FUNCTION_BLOCK "IMAC_TANK_CALL"
TITLE =Function calls for TANK objects
//Parameter Description for Function TANK (FB85):
//-----------------------------------------------
//OBJ:     Ascending Object number for TANK (1...x)
//
//XTsub:    'Substitution Value' for Tank Temperature. The value specified here
//          will be used instaed of the measured value, if the measured value is
//          invalid (Undefined or Out-of-Range or Faded Out or ObjNo invalid).
//          This value is only required, if the density compensation is 'ON' for
//          this tank (see Mode Switch M1_Temperature_Comp).
//          The Unit of XTsub is [°C]
//
//XDensity: 'Density' of the Medium in this tank.
//          This Value can be an input from OS or can be a fixed value.
//          The Unit of XDensity is [kg/dm3] or [tons/m3]
//
//XReftemp: 'Reference Temperature' for given density 'XDensity'.
//          This Value can be an input from OS or can be a fixed value.
//          This value is only required, if the density compensation is 'ON' for
//          this tank (see Mode Switch M1_Temperature_Comp).
//          The Unit of XRefTemp is [°C]
//
//XVEC:     'Volume Expansion Coefficient' - Change of density (staring from
//          XDensity at XReftemp) with every Kelvin of temperature change
//          This Value can be an input from OS or can be a fixed value.
//          This value is only required, if the density compensation is 'ON' for
//          this tank (see Mode Switch M1_Temperature_Comp).
//          The Unit of XVEC is [1/K]
//
//PCONF:    (leave empty, refers to local instance data in Instance DB)
//
//YVolume:  'Computed Volume' of Mediun in the tank
//          The Unit of YVolume is [m3]
//
//YMass:    'Computed Mass' of Mediun in the tank
//          The Unit of YMass is [tons]
//
//YLevel:   'Computed Level' of Mediun in the tank
//          The Unit of YLevel is [m]
//
//OSSTAT:   OS Status Word (not used for TANK)
//
//OSALARM:  OS Alarm Word  (not used for TANK)
//
//
//Units used in FB85 (TANK):
//Pressure MePo        : ................................... [Bar]
//Level MePo           : ................................... [m]
//Volume               : ................................... [m3]
//Temperature MePo     : ................................... [°C]
//Temperature Setpoint : ................................... [°C]
//Density              : ................................... [kg/dm3]
//Mass                 : ................................... [Tons]
//Vol.-Exp.Coefficient : ................................... [1/K]
AUTHOR : Edelmann
FAMILY : IMAC
VERSION : 0.1


VAR
  Tank_No001 : "IMAC_TANK";
  Tank_No002 : "IMAC_TANK";
  Tank_No003 : "IMAC_TANK";
  Tank_No004 : "IMAC_TANK";
  Tank_No005 : "IMAC_TANK";
  Tank_No006 : "IMAC_TANK";
  Tank_No007 : "IMAC_TANK";
  Tank_No008 : "IMAC_TANK";
  Tank_No009 : "IMAC_TANK";
  Tank_No010 : "IMAC_TANK";
END_VAR
BEGIN
NETWORK
TITLE =TANK Number 001

      CALL #Tank_No001 (
           OBJ                      := 1,
           XTsub                    := "IMAC_TANK_I/O".TANK_001_XTsub,// Temperature from OS or fixed value (Substitution Value, if Temp Sensor broken or not available)
           XDensity                 := "IMAC_TANK_I/O".TANK_001_XDensity,// Density from OS or fixed value
           XRefTemp                 := 2.000000e+001,// Reference Temperature for given Density value
           XVEC                     := 0.000000e+000,// Volume Expansion Coefficient from OS or fixed value
           YVolume                  := "IMAC_TANK_I/O".TANK_001_YVolume,// Computed Volume
           YMass                    := "IMAC_TANK_I/O".TANK_001_YMass,// Computed Mass
           YLevel                   := "IMAC_TANK_I/O".TANK_001_YLevel,// Computed Level
           OSSTAT                   := "IMAC_TANK_I/O".TANK_001_OSSTAT,// OS STATUS Word
           OSALARM                  := "IMAC_TANK_I/O".TANK_001_OSALARM);// OS ALARM Word

NETWORK
TITLE =TANK Number 002

//*********** END of function Processing ! *******************************************************************
      BEA   ; // Move this Instruction down to the next Network to add one object !
//************************************************************************************************************

      CALL #Tank_No002 (
           OBJ                      := 2,
           XTsub                    := "IMAC_TANK_I/O".TANK_002_XTsub,// Temperature from OS or fixed value (Substitution Value, if Temp Sensor broken or not available)
           XDensity                 := "IMAC_TANK_I/O".TANK_002_XDensity,// Density from OS or fixed value
           XRefTemp                 := 2.000000e+001,// Reference Temperature for given Density value
           XVEC                     := 0.000000e+000,// Volume Expansion Coefficient from OS or fixed value
           YVolume                  := "IMAC_TANK_I/O".TANK_002_YVolume,// Computed Volume
           YMass                    := "IMAC_TANK_I/O".TANK_002_YMass,// Computed Mass
           YLevel                   := "IMAC_TANK_I/O".TANK_002_YLevel,// Computed Level
           OSSTAT                   := "IMAC_TANK_I/O".TANK_002_OSSTAT,// OS STATUS Word
           OSALARM                  := "IMAC_TANK_I/O".TANK_002_OSALARM);// OS ALARM Word

NETWORK
TITLE =TANK Number 003

      CALL #Tank_No003 (
           OBJ                      := 3,
           XTsub                    := "IMAC_TANK_I/O".TANK_003_XTsub,// Temperature from OS or fixed value (Substitution Value, if Temp Sensor broken or not available)
           XDensity                 := "IMAC_TANK_I/O".TANK_003_XDensity,// Density from OS or fixed value
           XRefTemp                 := 2.000000e+001,// Reference Temperature for given Density value
           XVEC                     := 0.000000e+000,// Volume Expansion Coefficient from OS or fixed value
           YVolume                  := "IMAC_TANK_I/O".TANK_003_YVolume,// Computed Volume
           YMass                    := "IMAC_TANK_I/O".TANK_003_YMass,// Computed Mass
           YLevel                   := "IMAC_TANK_I/O".TANK_003_YLevel,// Computed Level
           OSSTAT                   := "IMAC_TANK_I/O".TANK_003_OSSTAT,// OS STATUS Word
           OSALARM                  := "IMAC_TANK_I/O".TANK_003_OSALARM);// OS ALARM Word

NETWORK
TITLE =TANK Number 004

      CALL #Tank_No004 (
           OBJ                      := 4,
           XTsub                    := "IMAC_TANK_I/O".TANK_004_XTsub,// Temperature from OS or fixed value (Substitution Value, if Temp Sensor broken or not available)
           XDensity                 := "IMAC_TANK_I/O".TANK_004_XDensity,// Density from OS or fixed value
           XRefTemp                 := 2.000000e+001,// Reference Temperature for given Density value
           XVEC                     := 0.000000e+000,// Volume Expansion Coefficient from OS or fixed value
           YVolume                  := "IMAC_TANK_I/O".TANK_004_YVolume,// Computed Volume
           YMass                    := "IMAC_TANK_I/O".TANK_004_YMass,// Computed Mass
           YLevel                   := "IMAC_TANK_I/O".TANK_004_YLevel,// Computed Level
           OSSTAT                   := "IMAC_TANK_I/O".TANK_004_OSSTAT,// OS STATUS Word
           OSALARM                  := "IMAC_TANK_I/O".TANK_004_OSALARM);// OS ALARM Word

NETWORK
TITLE =TANK Number 005

      CALL #Tank_No005 (
           OBJ                      := 5,
           XTsub                    := "IMAC_TANK_I/O".TANK_005_XTsub,// Temperature from OS or fixed value (Substitution Value, if Temp Sensor broken or not available)
           XDensity                 := "IMAC_TANK_I/O".TANK_005_XDensity,// Density from OS or fixed value
           XRefTemp                 := 2.000000e+001,// Reference Temperature for given Density value
           XVEC                     := 0.000000e+000,// Volume Expansion Coefficient from OS or fixed value
           YVolume                  := "IMAC_TANK_I/O".TANK_005_YVolume,// Computed Volume
           YMass                    := "IMAC_TANK_I/O".TANK_005_YMass,// Computed Mass
           YLevel                   := "IMAC_TANK_I/O".TANK_005_YLevel,// Computed Level
           OSSTAT                   := "IMAC_TANK_I/O".TANK_005_OSSTAT,// OS STATUS Word
           OSALARM                  := "IMAC_TANK_I/O".TANK_005_OSALARM);// OS ALARM Word

NETWORK
TITLE =TANK Number 006

      CALL #Tank_No006 (
           OBJ                      := 6,
           XTsub                    := "IMAC_TANK_I/O".TANK_006_XTsub,// Temperature from OS or fixed value (Substitution Value, if Temp Sensor broken or not available)
           XDensity                 := "IMAC_TANK_I/O".TANK_006_XDensity,// Density from OS or fixed value
           XRefTemp                 := 2.000000e+001,// Reference Temperature for given Density value
           XVEC                     := 0.000000e+000,// Volume Expansion Coefficient from OS or fixed value
           YVolume                  := "IMAC_TANK_I/O".TANK_006_YVolume,// Computed Volume
           YMass                    := "IMAC_TANK_I/O".TANK_006_YMass,// Computed Mass
           YLevel                   := "IMAC_TANK_I/O".TANK_006_YLevel,// Computed Level
           OSSTAT                   := "IMAC_TANK_I/O".TANK_006_OSSTAT,// OS STATUS Word
           OSALARM                  := "IMAC_TANK_I/O".TANK_006_OSALARM);// OS ALARM Word

NETWORK
TITLE =TANK Number 007

      CALL #Tank_No007 (
           OBJ                      := 7,
           XTsub                    := "IMAC_TANK_I/O".TANK_007_XTsub,// Temperature from OS or fixed value (Substitution Value, if Temp Sensor broken or not available)
           XDensity                 := "IMAC_TANK_I/O".TANK_007_XDensity,// Density from OS or fixed value
           XRefTemp                 := 2.000000e+001,// Reference Temperature for given Density value
           XVEC                     := 0.000000e+000,// Volume Expansion Coefficient from OS or fixed value
           YVolume                  := "IMAC_TANK_I/O".TANK_007_YVolume,// Computed Volume
           YMass                    := "IMAC_TANK_I/O".TANK_007_YMass,// Computed Mass
           YLevel                   := "IMAC_TANK_I/O".TANK_007_YLevel,// Computed Level
           OSSTAT                   := "IMAC_TANK_I/O".TANK_007_OSSTAT,// OS STATUS Word
           OSALARM                  := "IMAC_TANK_I/O".TANK_007_OSALARM);// OS ALARM Word

NETWORK
TITLE =TANK Number 008

      CALL #Tank_No008 (
           OBJ                      := 8,
           XTsub                    := "IMAC_TANK_I/O".TANK_008_XTsub,// Temperature from OS or fixed value (Substitution Value, if Temp Sensor broken or not available)
           XDensity                 := "IMAC_TANK_I/O".TANK_008_XDensity,// Density from OS or fixed value
           XRefTemp                 := 2.000000e+001,// Reference Temperature for given Density value
           XVEC                     := 0.000000e+000,// Volume Expansion Coefficient from OS or fixed value
           YVolume                  := "IMAC_TANK_I/O".TANK_008_YVolume,// Computed Volume
           YMass                    := "IMAC_TANK_I/O".TANK_008_YMass,// Computed Mass
           YLevel                   := "IMAC_TANK_I/O".TANK_008_YLevel,// Computed Level
           OSSTAT                   := "IMAC_TANK_I/O".TANK_008_OSSTAT,// OS STATUS Word
           OSALARM                  := "IMAC_TANK_I/O".TANK_008_OSALARM);// OS ALARM Word

NETWORK
TITLE =TANK Number 009

      CALL #Tank_No009 (
           OBJ                      := 9,
           XTsub                    := "IMAC_TANK_I/O".TANK_009_XTsub,// Temperature from OS or fixed value (Substitution Value, if Temp Sensor broken or not available)
           XDensity                 := "IMAC_TANK_I/O".TANK_009_XDensity,// Density from OS or fixed value
           XRefTemp                 := 2.000000e+001,// Reference Temperature for given Density value
           XVEC                     := 0.000000e+000,// Volume Expansion Coefficient from OS or fixed value
           YVolume                  := "IMAC_TANK_I/O".TANK_009_YVolume,// Computed Volume
           YMass                    := "IMAC_TANK_I/O".TANK_009_YMass,// Computed Mass
           YLevel                   := "IMAC_TANK_I/O".TANK_009_YLevel,// Computed Level
           OSSTAT                   := "IMAC_TANK_I/O".TANK_009_OSSTAT,// OS STATUS Word
           OSALARM                  := "IMAC_TANK_I/O".TANK_009_OSALARM);// OS ALARM Word

NETWORK
TITLE =TANK Number 010

      CALL #Tank_No010 (
           OBJ                      := 10,
           XTsub                    := "IMAC_TANK_I/O".TANK_010_XTsub,// Temperature from OS or fixed value (Substitution Value, if Temp Sensor broken or not available)
           XDensity                 := "IMAC_TANK_I/O".TANK_010_XDensity,// Density from OS or fixed value
           XRefTemp                 := 2.000000e+001,// Reference Temperature for given Density value
           XVEC                     := 0.000000e+000,// Volume Expansion Coefficient from OS or fixed value
           YVolume                  := "IMAC_TANK_I/O".TANK_010_YVolume,// Computed Volume
           YMass                    := "IMAC_TANK_I/O".TANK_010_YMass,// Computed Mass
           YLevel                   := "IMAC_TANK_I/O".TANK_010_YLevel,// Computed Level
           OSSTAT                   := "IMAC_TANK_I/O".TANK_010_OSSTAT,// OS STATUS Word
           OSALARM                  := "IMAC_TANK_I/O".TANK_010_OSALARM);// OS ALARM Word

END_FUNCTION_BLOCK

